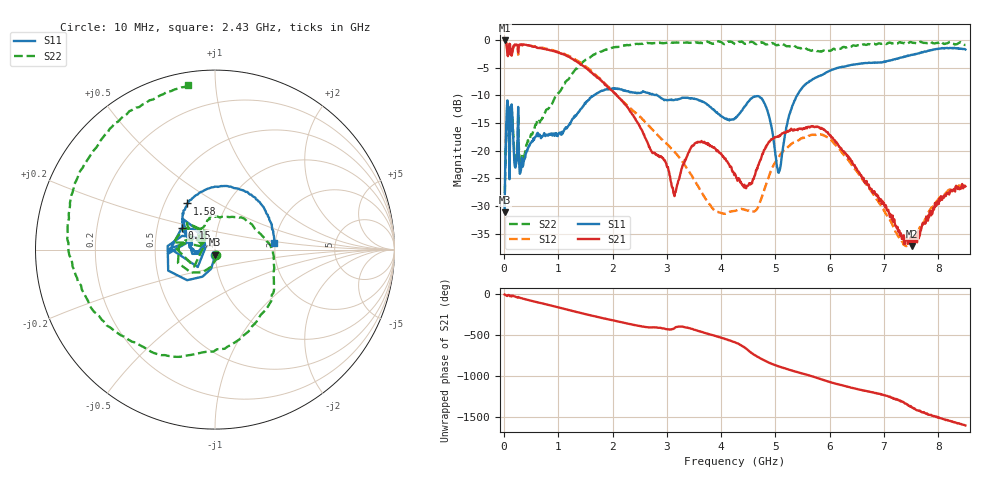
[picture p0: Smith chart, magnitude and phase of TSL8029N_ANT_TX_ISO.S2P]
!Agilent Technologies,E5071C,MY46523237,B.13.01
!Date: Wed Aug 16 14:00:35 2023
!Data & Calibration Information:
!Freq	S11:SOLT2(ON)	S21:SOLT2(ON)	S12:SOLT2(ON)	S22:SOLT2(ON)
!PortZ  Port1:50+j0  Port2:50+j0
!Above PortZ is port z conversion or system Z0 setting when saving the data.
!When reading, reference impedance value at option line is always used.
# Hz S dB R 50
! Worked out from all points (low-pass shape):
!   850 points, 10 MHz to 8.5 GHz, reference 50 ohm
!   highest |S21| = -0.04 dB at 10 MHz (marker M1); lowest = -37.2 dB at 7.52 GHz (marker M2)
!   |S21| within 3 dB of the highest: start of sweep to 1.203 GHz
!   lowest |S11| = -31.2 dB at 10 MHz (marker M3), VSWR 1.06, Z = 49.8 - j2.75 ohm
!   |S11| at or under -10 dB: start of sweep to 1.651 GHz; 2.826 GHz to 5.401 GHz (2.575 GHz wide, 62.6 % of centre)
!   |S22| runs from -29.9 to -0.2 dB; largest |S21 - S12| = 0.096
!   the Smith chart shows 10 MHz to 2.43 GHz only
!   S11 on the Smith chart (normalised r, x): 10 MHz: 1.00, -0.06; 150 MHz: 0.67, +0.17; 1.58 GHz: 0.65, +0.37; 2.43 GHz: 1.98, +0.17
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1e7  -31.16 -92.7  -0.04 -3.3  -0.05 -3.3  -29.95 -82.5
1.5e8  -13.11 146.5  -2.31 -16.2  -2.28 -20.3  -13.50 146.9
6.4e8  -17.05 169.6  -1.39 -101.9  -1.30 -101.2  -14.59 89.2
1.04e9  -16.70 152.8  -2.37 -167.4  -2.27 -166.2  -9.14 -20.5
1.43e9  -12.32 138.3  -4.43 127.5  -4.17 129.0  -4.19 -106.1
1.58e9  -10.47 120.8  -5.62 103.8  -5.32 104.6  -3.14 -134.2
1.98e9  -8.80 66.5  -9.06 44.2  -9.00 46.3  -1.39 160.6
2.43e9  -9.53 6.6  -14.50 -21.1  -13.18 -10.3  -0.65 99.2
2.84e9  -10.08 -53.2  -20.81 -50.3  -17.29 -58.7  -0.47 47.6
3.42e9  -10.49 -133.7  -19.83 -56.9  -23.96 -120.7  -0.47 -21.9
4.26e9  -14.06 23.5  -24.30 129.7  -30.89 -136.2  -0.71 -116.8
4.62e9  -10.23 -93.6  -24.51 -25.5  -30.95 -139.9  -0.63 -156.1
4.96e9  -17.60 141.7  -17.83 -141.1  -22.75 -154.0  -0.58 162.3
5.07e9  -23.71 42.2  -17.43 -167.3  -20.97 -173.8  -0.84 146.2
5.35e9  -10.92 -77.8  -16.30 134.8  -18.49 137.4  -1.03 103.2
5.67e9  -7.19 -130.1  -15.56 74.5  -17.14 78.3  -1.88 29.3
6.09e9  -5.18 -175.9  -18.09 -12.5  -18.78 -8.8  -1.62 -95.1
6.48e9  -4.34 145.7  -23.01 -78.0  -23.47 -75.6  -1.01 -178.0
7.09e9  -3.71 90.5  -31.29 -176.8  -32.25 -175.8  -0.44 103.6
7.52e9  -2.67 48.3  -37.22 50.9  -36.38 51.9  -0.45 61.8
8.04e9  -1.51 -20.4  -28.86 -80.2  -28.36 -79.9  -0.31 11.3
8.5e9  -1.67 -102.9  -26.45 -169.0  -26.32 -168.7  -0.85 -36.2
